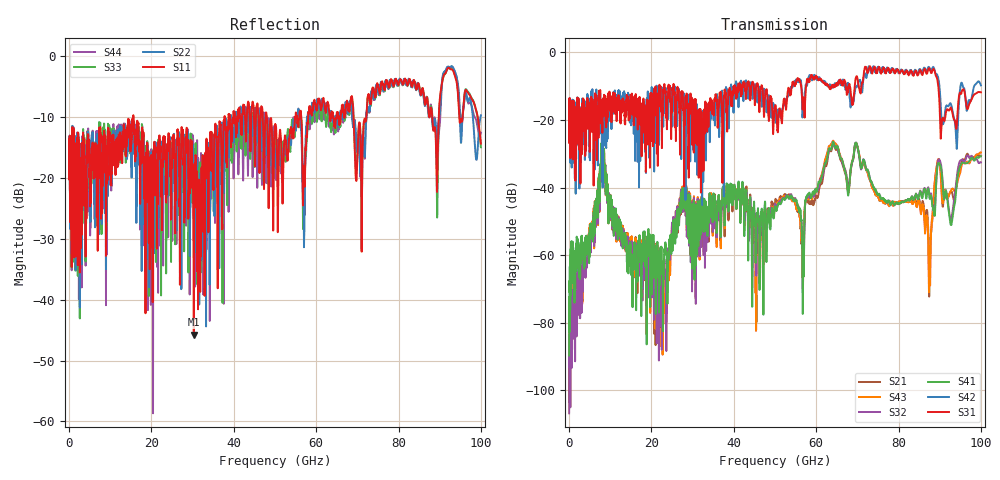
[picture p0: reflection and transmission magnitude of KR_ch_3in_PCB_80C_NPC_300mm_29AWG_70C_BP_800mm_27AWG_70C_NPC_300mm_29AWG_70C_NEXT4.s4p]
# GHz S RI R 45
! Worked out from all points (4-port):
!   4000 points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, 25 MHz to 100 GHz, reference 45 ohm
!   strongest paths, dB at 25 MHz, 25.02 GHz, 50.02 GHz, 75.03 GHz, 100 GHz:
!     S31: -20.0, -14.3, -16.2, -5.1, -11.8
!     S42: -20.0, -17.9, -18.0, -4.4, -9.7
!     S41: -89.7, -54.4, -45.6, -41.9, -30.7
!     S32: -106.8, -50.4, -44.9, -42.0, -32.5
!     S43: -102.7, -51.4, -44.8, -42.6, -29.6
!     S21: -103.5, -52.4, -44.7, -42.7, -30.6
!   lowest |S11| = -45.7 dB at 30.3 GHz (marker M1), VSWR 1.01, Z = 44.8 + j0.4 ohm
!   |S11| at or under -10 dB: start of sweep to 15.61 GHz; 15.64 GHz to 37.74 GHz (22.11 GHz wide, 82.8 % of centre); 48.04 GHz to 54.87 GHz (6.831 GHz wide, 13.3 % of centre)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
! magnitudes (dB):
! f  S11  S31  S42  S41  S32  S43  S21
! 25 MHz  -16.0  -20.0  -20.0  -89.7  -106.8  -102.7  -103.5
! 8.05 GHz  -17.1  -20.5  -23.6  -27.5  -28.2  -27.8  -27.9
! 23 GHz  -14.4  -12.1  -15.1  -66.2  -64.0  -68.8  -70.6
! 30.3 GHz  -45.7  -29.7  -20.1  -44.7  -43.6  -43.2  -43.5
! 64.28 GHz  -10.2  -10.3  -9.8  -26.9  -27.6  -26.4  -27.6
! 87.55 GHz  -9.9  -4.8  -4.7  -43.2  -42.9  -63.4  -60.9
! 100 GHz  -14.3  -11.8  -9.7  -30.7  -32.5  -29.6  -30.6
